FUNCTION_BLOCK FB_CSV
VAR_INPUT
	sPath: STRING(255);
	pRowData: ARRAY[1..MAX_CSV_COLUMNS] OF STRING(MAX_CSV_FIELD_LENGTH);
END_VAR
VAR_OUTPUT
	bRingBufferFull: BOOL;
END_VAR
VAR
	fbSysTime	: 	GETSYSTEMTIME;
	tFileTime	:	T_FILETIME;  
	
	_tNow		:	TIMESTRUCT; 
	   
	_iRowIndex: UDINT := 2; (*第1行存储字段名，2行存储PLC变量名*) 
	
	_iRingBuffer	: DWORD 	:= 0;
	
	fbFormat 	: 	FB_FormatString;
	_sPathFormat	: T_MaxString := '%s\%d__%d_%d_%d_%d_%d.csv';   
	_index: UDINT;
END_VAR
 
VAR CONSTANT
	cs_Seperator: STRING[1]:= ';'; (*CSV字段分隔符*)
	cs_CarriageReturn: STRING[2]:= '$R$N'; (*回车换行符*)
	
	MAX_BEFFER_SIZE:UINT := 8192;(*每条ADS写命令写下去的内存大小*)
END_VAR

fbSysTime(timeLoDW=>tFileTime.dwLowDateTime , timeHiDW=> tFileTime.dwHighDateTime);

_tNow := FILETIME_TO_SYSTEMTIME(tFileTime);
IF _tNow.wYear = 0 THEN
	RETURN;
END_IF
  
A_RowData();

_iRowIndex := _iRowIndex + 1;
IF _iRowIndex >= MAX_CSV_ROWS THEN 
	A_Header();	 	 
	gCSV_Buffer[_iRingBuffer].bFull := TRUE;
	
	fbFormat( 	sFormat := _sPathFormat ,
			 	arg1 := F_STRING(sPath),   arg2 := F_WORD(_tNow.wYear), arg3 := F_WORD(_tNow.wMonth), 
				arg4 := F_WORD(_tNow.wDay), arg5 := F_WORD(_tNow.wHour),arg6 := F_WORD(_tNow.wMinute),
			    arg7 := F_WORD(_tNow.wSecond),  sOut => gCSV_Buffer[_iRingBuffer].sPath);
				
	_iRingBuffer := _iRingBuffer + 1;
	IF _iRingBuffer > MAX_CSV_RING_BUFFER THEN
		IF gCSV_Buffer[_iRingBuffer].bFull THEN
			bRingBufferFull := TRUE;
		END_IF
		_iRingBuffer := 0; 
	END_IF
	_iRowIndex := 2;
END_IF

ACTION A_Header:
(*第一行 字段名称*) 
gCSV_Buffer[_iRingBuffer].aBuffer[ 0, 0] := 'WindSpeed';
gCSV_Buffer[_iRingBuffer].aBuffer[ 0, 1] := 'WindVane';
gCSV_Buffer[_iRingBuffer].aBuffer[ 0, 2] := 'TimeStampPLC3'; 
gCSV_Buffer[_iRingBuffer].aBuffer[ 0, 3] := 'TimeStampPLC4'; 
gCSV_Buffer[_iRingBuffer].aBuffer[ 0, 4] := 'TimeStampPLC5'; 

(*第二行 PLC变量名*)
gCSV_Buffer[_iRingBuffer].aBuffer[ 1, 0] := 'MAIN.var1';
gCSV_Buffer[_iRingBuffer].aBuffer[ 1, 1] := 'MAIN.var2'; 
gCSV_Buffer[_iRingBuffer].aBuffer[ 1, 2] := 'MAIN.var3'; 
gCSV_Buffer[_iRingBuffer].aBuffer[ 1, 3] := 'MAIN.var4'; 
gCSV_Buffer[_iRingBuffer].aBuffer[ 1, 4] := 'MAIN.var5';
END_ACTION

ACTION A_RowData:

(*数据行 从第三行开始*)


gCSV_Buffer[_iRingBuffer].aBuffer[_iRowIndex,0] := SYSTEMTIME_TO_STRING(_tNow);(*第二行第一列*)

FOR _index :=1 TO MAX_CSV_COLUMNS DO 
	gCSV_Buffer[_iRingBuffer].aBuffer[_iRowIndex,_index] := pRowData[_index];
END_FOR
END_ACTION

END_FUNCTION_BLOCK
